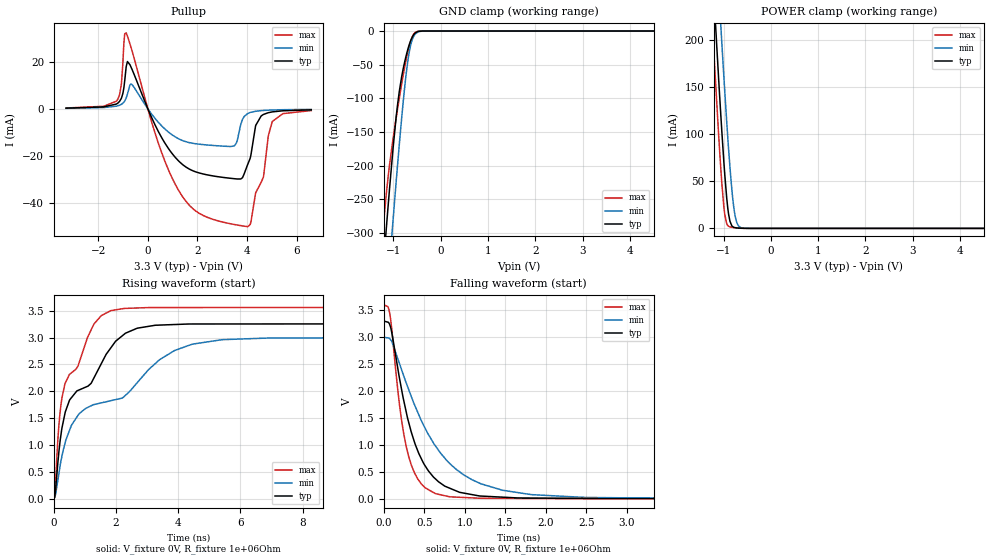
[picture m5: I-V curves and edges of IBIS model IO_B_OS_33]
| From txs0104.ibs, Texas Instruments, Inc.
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[Model]   IO_B_OS_33
Model_type   I/O_open_source
Polarity   Non-Inverting
Vinl=0.8
Vinh=2.0
Vmeas = 1.65
Vref = 0
Cref = 15pF
Rref = 1000
|   typ   min   max
C_comp   11.90pF   11.90pF   11.90pF
[Voltage Range]   3.3   3   3.6
[Temperature Range]   27   125   -40
[Pullup Reference]   3.3   3   3.6
[Pulldown Reference]   0   0   0
[Power Clamp Reference]   3.3   3   3.6
[GND Clamp Reference]   0   0   0
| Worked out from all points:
|   slope of the pullup table from 0 to 0.495 V, typ, clamps not added: 44.7 ohm
|   GND clamp passes 1 mA (typ) near -0.49 V on its own axis
|   POWER clamp passes 1 mA (typ) near -0.77 V on its own axis
|   falling waveform, V_fixture 0V, R_fixture 1e+06Ohm: 20-80 % time 342ps typ, 635ps min, 205ps max; typ from 3.3 V to 0 V
|   rising waveform, V_fixture 0V, R_fixture 1e+06Ohm: 20-80 % time 1.51ns typ, 2.84ns min, 921ps max; typ from 0 V to 3.3 V
[GND Clamp]
|   Voltage   I(typ)   I(min)   I(max)
-3.3V     -2.377A    -2.494A    -2.304A
-1.29V    -419.6mA   -539.1mA   -353.2mA
-1.211V   -347.3mA   -465.3mA   -287.2mA
-1.152V   -294.3mA   -410.5mA   -242.8mA
-1.082V   -234.6mA   -347.4mA   -199mA
-1.013V   -178.5mA   -285.5mA   -162.7mA
-914.1mV  -110.4mA   -200.2mA   -116.5mA
-825mV    -67.68mA   -128.7mA   -78.38mA
-676.5mV  -22.79mA   -36.04mA   -25.5mA
-607.2mV  -9.739mA   -14.07mA   -9.607mA
-528mV    -2.259mA   -3.768mA   -1.619mA
6.59V     0A         0A         0A
[Pullup]
|   Voltage   I(typ)   I(min)   I(max)
-3.3V     293.9uA    217.2uA    363.1uA
-1.261V   2.113mA    1.173mA    3.386mA
-1.073V   4.441mA    1.913mA    10.33mA
-874.5mV  18.03mA    4.63mA     32.41mA
-656.7mV  17.23mA    10.49mA    25.36mA
1.353V    -23.32mA   -13.31mA   -36.69mA
3.472V    -29.75mA   -15.84mA   -49.26mA
4.026V    -23.69mA   -2.005mA   -50.18mA
4.353V    -6.996mA   -1.017mA   -35.68mA
4.66V     -2.406mA   -686.5uA   -29.06mA
5.026V    -1.283mA   -492.4uA   -5.314mA
6.59V     -416.3uA   -221.4uA   -730.7uA
[POWER Clamp]
|   Voltage   I(typ)   I(min)   I(max)
-3.3V     2.284A     2.373A     2.231A
-1.261V   298.3mA    396.2mA    237.4mA
-1.211V   253.2mA    351mA      192.4mA
-1.191V   235.4mA    333mA      174.6mA
-1.102V   157.2mA    253.6mA    98.01mA
-1.043V   108.1mA    202.2mA    52.56mA
-973.5mV  56.77mA    144.8mA    14.55mA
-914.1mV  23.15mA    99.05mA    3.236mA
-864.6mV  7.565mA    64.86mA    1.581mA
-745.8mV  683.9uA    11.04mA    625.8uA
-597.3mV  119uA      420.7uA    82.08uA
6.59V     0A         0A         0A
[Ramp]
R_load = 1e+06
|   typ   min   max
dV/dt_r   1.97992/1.50865e-09   1.79687/2.84615e-09   2.15994/9.17305e-10
dV/dt_f   1.97992/3.43056e-10   1.79988/6.3394e-10   2.15994/2.04255e-10
[Falling Waveform]
V_fixture = 0V
V_fixture_min = 0V
V_fixture_max = 0V
R_fixture = 1e+06Ohm
C_fixture = 0F
|   Time   V(typ)   V(min)   V(max)
0s        3.3V       3V         3.6V
74.4ps    3.22V      2.966V     3.417V
213.9ps   2.062V     2.414V     1.498V
272.3ps   1.632V     2.162V     991.1mV
335.2ps   1.252V     1.91V      639.5mV
549.2ps   517.3mV    1.195V     168.1mV
809.7ps   196.8mV    658.8mV    36.33mV
1.468ns   28.31mV    156mV      6.214mV
2.492ns   5.289mV    23.06mV    1.178mV
19.9ns    0V         0V         0V
[Rising Waveform]
V_fixture = 0V
V_fixture_min = 0V
V_fixture_max = 0V
R_fixture = 1e+06Ohm
C_fixture = 0F
|   Time   V(typ)   V(min)   V(max)
0s        0V         5.026mV    0V
190.1ps   1.012V     565.9mV    1.544V
355.2ps   1.578V     1.02V      2.129V
823.8ps   2.027V     1.586V     2.55V
1.286ns   2.243V     1.751V     3.246V
1.834ns   2.808V     1.824V     3.5V
2.679ns   3.172V     2.157V     3.549V
3.879ns   3.241V     2.757V     3.558V
5.41ns    3.252V     2.959V     3.558V
19.9ns    3.3V       3V         3.6V
